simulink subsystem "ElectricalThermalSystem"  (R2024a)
settings: Solver=VariableStepAuto  StartTime=0.0  StopTime=10.0  RelTol=1e-3
undefined symbols (not defined in the file): EnvAirTemp, PlantThrEstCmpPwr, PlntThrAirBpt, PlntThrAirCond, PlntThrAirCp, PlntThrAirCpBpt, PlntThrAirPrand, PlntThrAirRho, PlntThrAirVisc, PlntThrBattDCFlwRatio, PlntThrBattJacLen, PlntThrChArea, PlntThrChDia, PlntThrCoolCond, PlntThrCoolCp, PlntThrCoolCpBpt, PlntThrCoolPrand, PlntThrCoolRho, PlntThrCoolVisc, PlntThrDCJacLen, PlntThrEMJacLen, PlntThrEstCOPLut, PlntThrEstDTLut, PlntThrHeaterMaxPwr, PlntThrPmpDisp, PlntThrPmpHeadP, PlntThrPmpMaxSpd, PlntThrPmpMechEff, PlntThrPmpVolEff, PlntThrRadAirArea, PlntThrRadAirDh, PlntThrRadFanAreaFlw, PlntThrRadFlwCoef, PlntThrRadGapHeight, PlntThrRadLength, PlntThrRadNTubes, PlntThrRadTubeDh, PlntThrRadTubeHeight, PlntThrRadWidth
libraries: autolibutils x45
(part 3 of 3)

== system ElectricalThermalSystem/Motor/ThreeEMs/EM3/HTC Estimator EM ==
  FluidTemp : Inport
  MassFlow : Inport  Port=2
  CrossA : Inport  Port=3  OutMin=eps
  HydDia : Inport  Port=4
  TubLen : Inport  Port=5
  Abs Viscosity : Lookup_n-D  NumberOfTableDimensions=1  BreakpointsForDimension1=PlntThrCoolCpBpt  Table=PlntThrCoolVisc  ExtrapMethod=Clip  UseLastTableValue=on  InternalRulePriority=Speed  RndMeth=Simplest
  Calculation1 : Fcn  Expr=u(1)^0.8*u(2)^0.33
  Calculation2 : Fcn  Expr=0.036*u(1)*u(2)^0.055
  Divide : Product  Inputs=**//
  Divide2 : Product  Inputs=*/
  Divide3 : Product  Inputs=*/
  Gain : Gain  Gain=0.023
  Math Function : Math  Operator=reciprocal
  Prandtl Number : Lookup_n-D  NumberOfTableDimensions=1  BreakpointsForDimension1=PlntThrCoolCpBpt  Table=PlntThrCoolPrand  ExtrapMethod=Clip  UseLastTableValue=on  InternalRulePriority=Speed  RndMeth=Simplest
  Product1 : Product
  Switch5 : Switch  Threshold=400
  Thermal Conductivity : Lookup_n-D  NumberOfTableDimensions=1  BreakpointsForDimension1=PlntThrCoolCpBpt  Table=PlntThrCoolCond  ExtrapMethod=Clip  UseLastTableValue=on  InternalRulePriority=Speed  RndMeth=Simplest
  Transfer Fcn1 : TransferFcn  Denominator=[0.1 1]
  Vector Concatenate : Concatenate
  Vector Concatenate1 : Concatenate
  HTC : Outport
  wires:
  Transfer Fcn1/1 -> HTC/1  "HTCest"
  FluidTemp/1 -> Prandtl Number/1, [CoolTemp], Abs Viscosity/1
  [CoolTemp] -> Thermal Conductivity/1
  MassFlow/1 -> Divide/1
  HydDia/1 -> [HydD], Divide/2
  CrossA/1 -> Divide/3
  [HydD] -> Divide2/1
  TubLen/1 -> Divide2/2
  Divide2/1 -> [DoL]
  Abs Viscosity/1 -> Divide/4
  Divide/1 -> Vector Concatenate1/1  "ReD"
  Prandtl Number/1 -> Vector Concatenate1/2
  Vector Concatenate1/1 -> Calculation1/1
  [DoL] -> Math Function/1
  Math Function/1 -> Switch5/2
  Thermal Conductivity/1 -> Divide3/1
  [HydD] -> Divide3/2
  Divide3/1 -> Product1/1
  Gain/1 -> Switch5/1
  Calculation1/1 -> [RePr], Gain/1
  [RePr] -> Vector Concatenate/1
  [DoL] -> Vector Concatenate/2
  Vector Concatenate/1 -> Calculation2/1
  Calculation2/1 -> Switch5/3
  Switch5/1 -> Product1/2  "NuD"
  Product1/1 -> Transfer Fcn1/1

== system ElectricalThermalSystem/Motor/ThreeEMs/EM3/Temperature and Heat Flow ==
  HTC : Inport
  CoolTempIn : Inport  Port=2
  EMTemp : Inport  Port=3
  CoolMflw : Inport  Port=4
  JacArea : Inport  Port=5
  Divide2 : Product  Inputs=*/
  Gain4 : Gain  Gain=0.5
  LPF with IC1 : Subsystem  mask{wc=10, InitCond=EnvAirTemp, dataType=off}
      mask prompts: wc "Cutoff frequency, wc [rad/s]"; InitCond "Initial condition, InitCond [same as u]"; dataType "Enforce same input data type"
  Minus3 : Sum
  Minus4 : Sum
  Product1 : Product  Inputs=3
  Product2 : Product
  Selector : Selector  InputPortWidth=PlntEMNum  IndexOptions=Index vector (dialog)  Indices=3  OutputSizes=1
  Specific Heat 2 : Lookup_n-D  NumberOfTableDimensions=1  BreakpointsForDimension1=PlntThrCoolCpBpt  Table=PlntThrCoolCp  ExtrapMethod=Clip  UseLastTableValue=on  InternalRulePriority=Speed  RndMeth=Simplest
  Subtract : Sum  Inputs=+-
  div0protect - abs poly4 : autolibutils/div0protect - abs poly  thresh=.001  aMode=1
  BulkCoolTemp : Outport
  Qem : Outport  Port=2
  CoolTempOut : Outport  Port=3
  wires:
  LPF with IC1/1(y) -> BulkCoolTemp/1, [BulkCoolTemp]
  EMTemp/1 -> Selector/1
  HTC/1 -> Product1/1
  Product2/1 -> div0protect - abs poly4/1
  Minus4/1 -> Gain4/1
  Gain4/1 -> LPF with IC1/1(u)
  Minus3/1 -> Minus4/2, CoolTempOut/1
  Product1/1 -> Divide2/1, Qem/1  "Qem"
  JacArea/1 -> Product1/2
  div0protect - abs poly4/1 -> Divide2/2
  Specific Heat 2/1 -> Product2/2
  [BulkCoolTemp] -> Specific Heat 2/1, Subtract/2
  Subtract/1 -> Product1/3
  Selector/1 -> Subtract/1
  Divide2/1 -> Minus3/2
  CoolMflw/1 -> Product2/1
  CoolTempIn/1 -> Minus4/1, Minus3/1

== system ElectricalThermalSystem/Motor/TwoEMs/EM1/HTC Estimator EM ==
  FluidTemp : Inport
  MassFlow : Inport  Port=2
  CrossA : Inport  Port=3  OutMin=eps
  HydDia : Inport  Port=4
  TubLen : Inport  Port=5
  Abs Viscosity : Lookup_n-D  NumberOfTableDimensions=1  BreakpointsForDimension1=PlntThrCoolCpBpt  Table=PlntThrCoolVisc  ExtrapMethod=Clip  UseLastTableValue=on  InternalRulePriority=Speed  RndMeth=Simplest
  Calculation1 : Fcn  Expr=u(1)^0.8*u(2)^0.33
  Calculation2 : Fcn  Expr=0.036*u(1)*u(2)^0.055
  Divide : Product  Inputs=**//
  Divide2 : Product  Inputs=*/
  Divide3 : Product  Inputs=*/
  Gain : Gain  Gain=0.023
  Math Function : Math  Operator=reciprocal
  Prandtl Number : Lookup_n-D  NumberOfTableDimensions=1  BreakpointsForDimension1=PlntThrCoolCpBpt  Table=PlntThrCoolPrand  ExtrapMethod=Clip  UseLastTableValue=on  InternalRulePriority=Speed  RndMeth=Simplest
  Product1 : Product
  Switch5 : Switch  Threshold=400
  Thermal Conductivity : Lookup_n-D  NumberOfTableDimensions=1  BreakpointsForDimension1=PlntThrCoolCpBpt  Table=PlntThrCoolCond  ExtrapMethod=Clip  UseLastTableValue=on  InternalRulePriority=Speed  RndMeth=Simplest
  Transfer Fcn1 : TransferFcn  Denominator=[0.1 1]
  Vector Concatenate : Concatenate
  Vector Concatenate1 : Concatenate
  HTC : Outport
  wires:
  Transfer Fcn1/1 -> HTC/1  "HTCest"
  FluidTemp/1 -> Prandtl Number/1, [CoolTemp], Abs Viscosity/1
  [CoolTemp] -> Thermal Conductivity/1
  MassFlow/1 -> Divide/1
  HydDia/1 -> [HydD], Divide/2
  CrossA/1 -> Divide/3
  [HydD] -> Divide2/1
  TubLen/1 -> Divide2/2
  Divide2/1 -> [DoL]
  Abs Viscosity/1 -> Divide/4
  Divide/1 -> Vector Concatenate1/1  "ReD"
  Prandtl Number/1 -> Vector Concatenate1/2
  Vector Concatenate1/1 -> Calculation1/1
  [DoL] -> Math Function/1
  Math Function/1 -> Switch5/2
  Thermal Conductivity/1 -> Divide3/1
  [HydD] -> Divide3/2
  Divide3/1 -> Product1/1
  Gain/1 -> Switch5/1
  Calculation1/1 -> [RePr], Gain/1
  [RePr] -> Vector Concatenate/1
  [DoL] -> Vector Concatenate/2
  Vector Concatenate/1 -> Calculation2/1
  Calculation2/1 -> Switch5/3
  Switch5/1 -> Product1/2  "NuD"
  Product1/1 -> Transfer Fcn1/1

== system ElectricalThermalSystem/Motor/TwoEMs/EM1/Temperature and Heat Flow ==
  HTC : Inport
  CoolTempIn : Inport  Port=2
  EMTemp : Inport  Port=3
  CoolMflw : Inport  Port=4
  JacArea : Inport  Port=5
  Divide2 : Product  Inputs=*/
  Gain4 : Gain  Gain=0.5
  LPF with IC1 : Subsystem  mask{wc=10, InitCond=EnvAirTemp, dataType=off}
      mask prompts: wc "Cutoff frequency, wc [rad/s]"; InitCond "Initial condition, InitCond [same as u]"; dataType "Enforce same input data type"
  Minus3 : Sum
  Minus4 : Sum
  Product1 : Product  Inputs=3
  Product2 : Product
  Selector : Selector  InputPortWidth=PlntEMNum  IndexOptions=Index vector (dialog)  Indices=1  OutputSizes=1
  Specific Heat 2 : Lookup_n-D  NumberOfTableDimensions=1  BreakpointsForDimension1=PlntThrCoolCpBpt  Table=PlntThrCoolCp  ExtrapMethod=Clip  UseLastTableValue=on  InternalRulePriority=Speed  RndMeth=Simplest
  Subtract : Sum  Inputs=+-
  div0protect - abs poly4 : autolibutils/div0protect - abs poly  thresh=.001  aMode=1
  BulkCoolTemp : Outport
  Qem : Outport  Port=2
  CoolTempOut : Outport  Port=3
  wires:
  LPF with IC1/1(y) -> BulkCoolTemp/1, [BulkCoolTemp]
  EMTemp/1 -> Selector/1
  HTC/1 -> Product1/1
  Product2/1 -> div0protect - abs poly4/1
  Minus4/1 -> Gain4/1
  Gain4/1 -> LPF with IC1/1(u)
  Minus3/1 -> Minus4/2, CoolTempOut/1
  Product1/1 -> Divide2/1, Qem/1  "Qem"
  JacArea/1 -> Product1/2
  div0protect - abs poly4/1 -> Divide2/2
  Specific Heat 2/1 -> Product2/2
  [BulkCoolTemp] -> Specific Heat 2/1, Subtract/2
  Subtract/1 -> Product1/3
  Selector/1 -> Subtract/1
  Divide2/1 -> Minus3/2
  CoolMflw/1 -> Product2/1
  CoolTempIn/1 -> Minus4/1, Minus3/1

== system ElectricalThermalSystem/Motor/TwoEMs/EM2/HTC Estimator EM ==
  FluidTemp : Inport
  MassFlow : Inport  Port=2
  CrossA : Inport  Port=3  OutMin=eps
  HydDia : Inport  Port=4
  TubLen : Inport  Port=5
  Abs Viscosity : Lookup_n-D  NumberOfTableDimensions=1  BreakpointsForDimension1=PlntThrCoolCpBpt  Table=PlntThrCoolVisc  ExtrapMethod=Clip  UseLastTableValue=on  InternalRulePriority=Speed  RndMeth=Simplest
  Calculation1 : Fcn  Expr=u(1)^0.8*u(2)^0.33
  Calculation2 : Fcn  Expr=0.036*u(1)*u(2)^0.055
  Divide : Product  Inputs=**//
  Divide2 : Product  Inputs=*/
  Divide3 : Product  Inputs=*/
  Gain : Gain  Gain=0.023
  Math Function : Math  Operator=reciprocal
  Prandtl Number : Lookup_n-D  NumberOfTableDimensions=1  BreakpointsForDimension1=PlntThrCoolCpBpt  Table=PlntThrCoolPrand  ExtrapMethod=Clip  UseLastTableValue=on  InternalRulePriority=Speed  RndMeth=Simplest
  Product1 : Product
  Switch5 : Switch  Threshold=400
  Thermal Conductivity : Lookup_n-D  NumberOfTableDimensions=1  BreakpointsForDimension1=PlntThrCoolCpBpt  Table=PlntThrCoolCond  ExtrapMethod=Clip  UseLastTableValue=on  InternalRulePriority=Speed  RndMeth=Simplest
  Transfer Fcn1 : TransferFcn  Denominator=[0.1 1]
  Vector Concatenate : Concatenate
  Vector Concatenate1 : Concatenate
  HTC : Outport
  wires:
  Transfer Fcn1/1 -> HTC/1  "HTCest"
  FluidTemp/1 -> Prandtl Number/1, [CoolTemp], Abs Viscosity/1
  [CoolTemp] -> Thermal Conductivity/1
  MassFlow/1 -> Divide/1
  HydDia/1 -> [HydD], Divide/2
  CrossA/1 -> Divide/3
  [HydD] -> Divide2/1
  TubLen/1 -> Divide2/2
  Divide2/1 -> [DoL]
  Abs Viscosity/1 -> Divide/4
  Divide/1 -> Vector Concatenate1/1  "ReD"
  Prandtl Number/1 -> Vector Concatenate1/2
  Vector Concatenate1/1 -> Calculation1/1
  [DoL] -> Math Function/1
  Math Function/1 -> Switch5/2
  Thermal Conductivity/1 -> Divide3/1
  [HydD] -> Divide3/2
  Divide3/1 -> Product1/1
  Gain/1 -> Switch5/1
  Calculation1/1 -> [RePr], Gain/1
  [RePr] -> Vector Concatenate/1
  [DoL] -> Vector Concatenate/2
  Vector Concatenate/1 -> Calculation2/1
  Calculation2/1 -> Switch5/3
  Switch5/1 -> Product1/2  "NuD"
  Product1/1 -> Transfer Fcn1/1

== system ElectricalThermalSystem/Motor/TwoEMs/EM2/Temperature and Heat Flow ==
  HTC : Inport
  CoolTempIn : Inport  Port=2
  EMTemp : Inport  Port=3
  CoolMflw : Inport  Port=4
  JacArea : Inport  Port=5
  Divide2 : Product  Inputs=*/
  Gain4 : Gain  Gain=0.5
  LPF with IC1 : Subsystem  mask{wc=10, InitCond=EnvAirTemp, dataType=off}
      mask prompts: wc "Cutoff frequency, wc [rad/s]"; InitCond "Initial condition, InitCond [same as u]"; dataType "Enforce same input data type"
  Minus3 : Sum
  Minus4 : Sum
  Product1 : Product  Inputs=3
  Product2 : Product
  Selector : Selector  InputPortWidth=PlntEMNum  IndexOptions=Index vector (dialog)  Indices=2  OutputSizes=1
  Specific Heat 2 : Lookup_n-D  NumberOfTableDimensions=1  BreakpointsForDimension1=PlntThrCoolCpBpt  Table=PlntThrCoolCp  ExtrapMethod=Clip  UseLastTableValue=on  InternalRulePriority=Speed  RndMeth=Simplest
  Subtract : Sum  Inputs=+-
  div0protect - abs poly4 : autolibutils/div0protect - abs poly  thresh=.001  aMode=1
  BulkCoolTemp : Outport
  Qem : Outport  Port=2
  CoolTempOut : Outport  Port=3
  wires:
  LPF with IC1/1(y) -> BulkCoolTemp/1, [BulkCoolTemp]
  EMTemp/1 -> Selector/1
  HTC/1 -> Product1/1
  Product2/1 -> div0protect - abs poly4/1
  Minus4/1 -> Gain4/1
  Gain4/1 -> LPF with IC1/1(u)
  Minus3/1 -> Minus4/2, CoolTempOut/1
  Product1/1 -> Divide2/1, Qem/1  "Qem"
  JacArea/1 -> Product1/2
  div0protect - abs poly4/1 -> Divide2/2
  Specific Heat 2/1 -> Product2/2
  [BulkCoolTemp] -> Specific Heat 2/1, Subtract/2
  Subtract/1 -> Product1/3
  Selector/1 -> Subtract/1
  Divide2/1 -> Minus3/2
  CoolMflw/1 -> Product2/1
  CoolTempIn/1 -> Minus4/1, Minus3/1

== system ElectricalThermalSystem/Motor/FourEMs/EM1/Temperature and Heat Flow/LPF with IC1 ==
  u : Inport
  Cont LPF IC : autolibutils/Cont LPF IC  wc=wc  aMode=1  dataType=off
  Initial Condition : Constant  Value=InitCond  SampleTime=-1
  y : Outport
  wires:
  Cont LPF IC/1 -> y/1
  u/1 -> Cont LPF IC/1
  Initial Condition/1 -> Cont LPF IC/2

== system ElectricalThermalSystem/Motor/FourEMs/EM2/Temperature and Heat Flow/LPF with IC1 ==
  u : Inport
  Cont LPF IC : autolibutils/Cont LPF IC  wc=wc  aMode=1  dataType=off
  Initial Condition : Constant  Value=InitCond  SampleTime=-1
  y : Outport
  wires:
  Cont LPF IC/1 -> y/1
  u/1 -> Cont LPF IC/1
  Initial Condition/1 -> Cont LPF IC/2

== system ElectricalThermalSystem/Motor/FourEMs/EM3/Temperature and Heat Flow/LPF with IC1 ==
  u : Inport
  Cont LPF IC : autolibutils/Cont LPF IC  wc=wc  aMode=1  dataType=off
  Initial Condition : Constant  Value=InitCond  SampleTime=-1
  y : Outport
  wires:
  Cont LPF IC/1 -> y/1
  u/1 -> Cont LPF IC/1
  Initial Condition/1 -> Cont LPF IC/2

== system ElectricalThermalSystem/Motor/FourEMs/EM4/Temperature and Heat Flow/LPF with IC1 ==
  u : Inport
  Cont LPF IC : autolibutils/Cont LPF IC  wc=wc  aMode=1  dataType=off
  Initial Condition : Constant  Value=InitCond  SampleTime=-1
  y : Outport
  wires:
  Cont LPF IC/1 -> y/1
  u/1 -> Cont LPF IC/1
  Initial Condition/1 -> Cont LPF IC/2

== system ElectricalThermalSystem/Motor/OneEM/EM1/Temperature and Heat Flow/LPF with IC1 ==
  u : Inport
  Cont LPF IC : autolibutils/Cont LPF IC  wc=wc  aMode=1  dataType=off
  Initial Condition : Constant  Value=InitCond  SampleTime=-1
  y : Outport
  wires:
  Cont LPF IC/1 -> y/1
  u/1 -> Cont LPF IC/1
  Initial Condition/1 -> Cont LPF IC/2

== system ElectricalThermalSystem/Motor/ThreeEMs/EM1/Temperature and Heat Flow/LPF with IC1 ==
  u : Inport
  Cont LPF IC : autolibutils/Cont LPF IC  wc=wc  aMode=1  dataType=off
  Initial Condition : Constant  Value=InitCond  SampleTime=-1
  y : Outport
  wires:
  Cont LPF IC/1 -> y/1
  u/1 -> Cont LPF IC/1
  Initial Condition/1 -> Cont LPF IC/2

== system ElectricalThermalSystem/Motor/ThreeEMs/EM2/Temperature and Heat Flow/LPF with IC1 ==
  u : Inport
  Cont LPF IC : autolibutils/Cont LPF IC  wc=wc  aMode=1  dataType=off
  Initial Condition : Constant  Value=InitCond  SampleTime=-1
  y : Outport
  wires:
  Cont LPF IC/1 -> y/1
  u/1 -> Cont LPF IC/1
  Initial Condition/1 -> Cont LPF IC/2

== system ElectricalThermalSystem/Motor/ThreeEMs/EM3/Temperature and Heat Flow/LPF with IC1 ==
  u : Inport
  Cont LPF IC : autolibutils/Cont LPF IC  wc=wc  aMode=1  dataType=off
  Initial Condition : Constant  Value=InitCond  SampleTime=-1
  y : Outport
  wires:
  Cont LPF IC/1 -> y/1
  u/1 -> Cont LPF IC/1
  Initial Condition/1 -> Cont LPF IC/2

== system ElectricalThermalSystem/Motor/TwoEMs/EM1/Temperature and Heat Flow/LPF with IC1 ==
  u : Inport
  Cont LPF IC : autolibutils/Cont LPF IC  wc=wc  aMode=1  dataType=off
  Initial Condition : Constant  Value=InitCond  SampleTime=-1
  y : Outport
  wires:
  Cont LPF IC/1 -> y/1
  u/1 -> Cont LPF IC/1
  Initial Condition/1 -> Cont LPF IC/2

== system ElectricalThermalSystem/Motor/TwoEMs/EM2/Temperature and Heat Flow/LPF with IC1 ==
  u : Inport
  Cont LPF IC : autolibutils/Cont LPF IC  wc=wc  aMode=1  dataType=off
  Initial Condition : Constant  Value=InitCond  SampleTime=-1
  y : Outport
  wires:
  Cont LPF IC/1 -> y/1
  u/1 -> Cont LPF IC/1
  Initial Condition/1 -> Cont LPF IC/2
